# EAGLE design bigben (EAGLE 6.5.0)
AUTHOR: Brad Campbell; REV: A; TITLE: BigBen
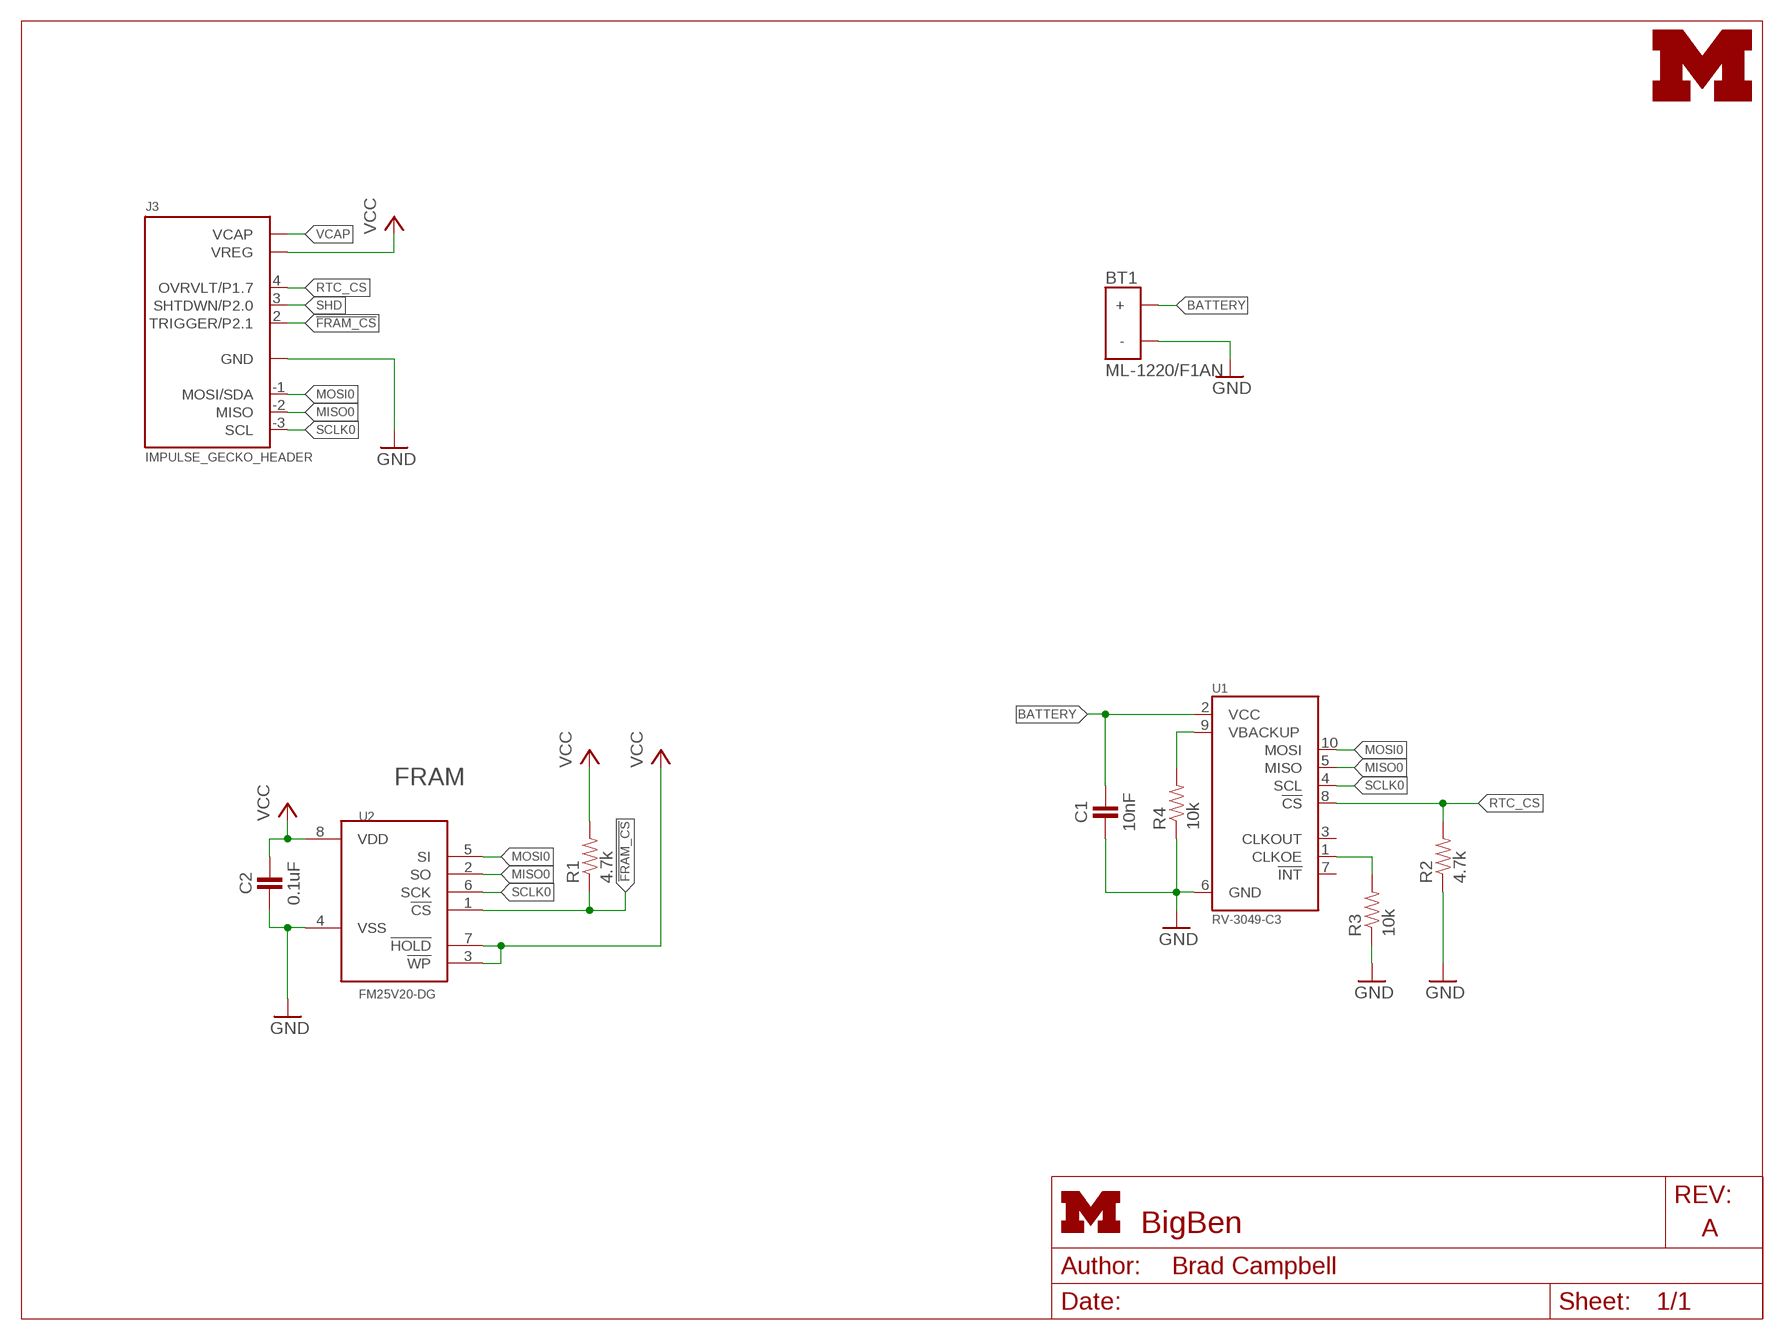
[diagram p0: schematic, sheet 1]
FRAME1 (LETTER_L): HEIGHT: 8.5in; WIDTH: 11in

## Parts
BT1  ML-1220/F1AN  [ML-1220/F1BN]
C1  10nF  CAPACITOR  [0402_CAP]
C2  0.1uF  CAPACITOR  [0402_CAP]
J3  IMPULSE_GECKO_HEADER  [HEADER1X9/0.05IN]
LOGO1  UMICH_SOLID_TINY  [UMICH_SOLID_50MIL]
R1  4.7k  RESISTOR  [0402_RES]
R2  4.7k  RESISTOR  [0402_RES]
R3  10k  RESISTOR  [0402_RES]
R4  10k  RESISTOR  [0402_RES]
U1  RV-3049-C3  [MICRO-CRYSTAL-C3]
U2  FM25V20-DG  [TDFN-8/6MM]

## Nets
!FRAM_CS: J3.2(TRIGGER/P2.1) R1.1 U2.1(!CS)
BATTERY: BT1.POS(+) C1.1 U1.2(VCC)
GND: BT1.NEG(-) C1.2 C2.2 J3.0(GND) R2.1 R3.1 R4.1 U1.6(GND) U2.4(VSS)
MISO0: J3.-2(MISO) U1.5(MISO) U2.2(SO)
MOSI0: J3.-1(MOSI/SDA) U1.10(MOSI) U2.5(SI)
N$6: R4.2 U1.9(VBACKUP)
N$7: R3.2 U1.1(CLKOE)
RTC_CS: J3.4(OVRVLT/P1.7) R2.2 U1.8(!CS)
SCLK0: J3.-3(SCL) U1.4(SCL) U2.6(SCK)
SHD: J3.3(SHTDWN/P2.0)
VCAP: J3.5(VCAP)
VCC: C2.1 J3.1(VREG) R1.2 U2.3(!WP) U2.7(!HOLD) U2.8(VDD)
Unconnected: U1.3(CLKOUT) U1.7(!INT)

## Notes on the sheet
- FRAM

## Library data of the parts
BT1 = batteries:ML-1220/F1AN: BATTERY LITH 3V RECHARGE PC PINS; DIGIKEY: P663-nd; MOUSER: 658-ML-1220/F1BN
C1 C2 = passives:CAPACITOR: 0402 Capacitor
J3 = gecko:IMPULSE_GECKO_HEADER: Header on the impulse EPIC-esque board.
LOGO1 = logos:UMICH_SOLID
R1-R4 = passives:RESISTOR: Resistor
U1 = chips:RV-3049-C3: The RV-3049-C3 is an ultra miniature Real-Time-Clock Module with embedded Crystal. This RTC has an SPI Bus (4-wire Serial- Interface) and offers temperature compensated time.
U2 = chips:FM25: Cypress FRAM; DIGIKEY: FM25V20-DGRA-ND; MOUSER: 877-FM25V20-DG

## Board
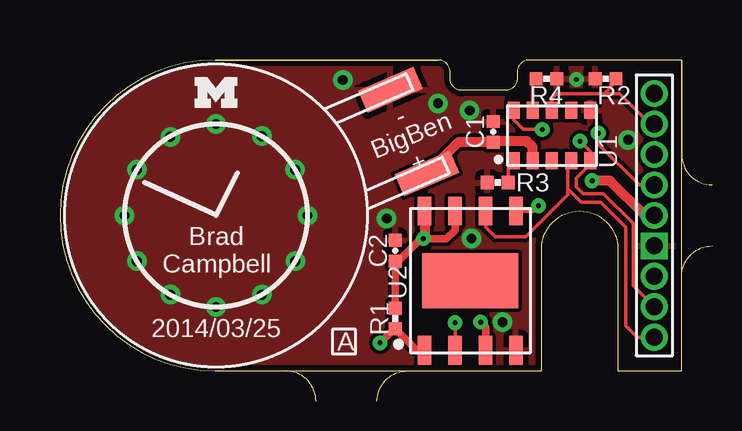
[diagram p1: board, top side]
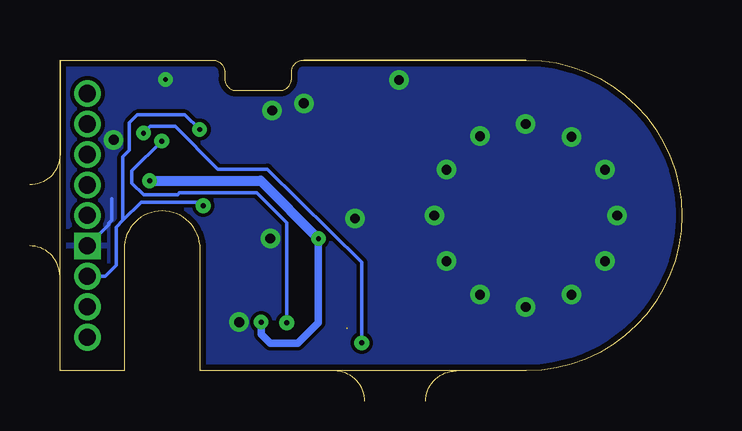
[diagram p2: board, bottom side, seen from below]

Size 25.91 x 12.95 mm. Coordinates in mm from the lower left corner, seen from the top.
Outline: 6.48,0 20.07,0 20.07,5.08 arc-180 23.24,5.08 23.24,0 25.91,0 25.91,12.95 19.56,12.95 arc90 19.05,12.45 19.05,12.19 arc-90 18.54,11.68 16.76,11.68 arc-90 16.26,12.19 16.26,12.45 arc90 15.75,12.95 6.48,12.95 arc180 6.48,0
Copper layers (1*16): Top 0.0178mm / dielectric 59mil / Bottom 0.0178mm
Design rules "sunstone-2lyr_v1.0.0.3 *": minimum track width 6mil, minimum drill 14mil, track to track 6mil, track to pad 6mil, pad to pad 6mil, via to via 6mil, smd to smd 6mil, copper to edge 10mil, drill to drill 16mil, minimum pad ring 8mil, minimum via ring 8mil, stop-mask expansion 3mil, vias tented up to drill 100mil, thermal gap 10mil
Milling: 22 lines

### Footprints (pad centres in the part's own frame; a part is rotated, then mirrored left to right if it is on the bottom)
ML-1220/F1BN = smd 2.5 x 1: NEG 8.75,1.9; POS 8.75,-1.9
0402_CAP = smd 0.536 x 0.546: 1 -0.433,0; 2 0.433,0
HEADER1X9/0.05IN = drill 0.711 pad 1.016 square: 0 -1.27,0 | drill 0.711 pad 1.016: 1 0,0; 2 1.27,0; 3 2.54,0; 4 3.81,0; 5 5.08,0; -1 -2.54,0; -2 -3.81,0; -3 -5.08,0
0402_RES = smd 0.536 x 0.546: 1 -0.433,0; 2 0.433,0
MICRO-CRYSTAL-C3 = smd 0.5 x 0.7: 1 -1.6,-1.05; 2 -0.8,-1.05; 3 0,-1.05; 4 0.8,-1.05; 5 1.6,-1.05; 6 1.6,1.05; 7 0.8,1.05; 8 0,1.05; 9 -0.8,1.05; 10 -1.6,1.05
TDFN-8/6MM = smd 0.55 x 1.2: 1 -1.905,-2.9; 2 -0.635,-2.9; 3 0.635,-2.9; 4 1.905,-2.9; 5 1.905,2.9; 6 0.635,2.9; 7 -0.635,2.9; 8 -1.905,2.9 | smd 4 x 2.3: NC 0,0

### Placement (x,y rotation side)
BT1  6.5,6.48 23.5 top
C1  18.06,9.96 90 top
C2  13.97,5 90 top
J3  24.77,6.48 90 top
LOGO1  6.5,11.61 0 top
R1  13.97,2.18 90 top
R2  22.73,12.17 0 top
R3  18.24,7.85 0 top
R4  20.27,12.17 180 top
U1  20.5,9.8 0 top
U2  17.09,3.76 0 top

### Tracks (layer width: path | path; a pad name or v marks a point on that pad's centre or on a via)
!FRAM_CS  (via drill 0.2)  (1 unrouted)
  Top 0.152: J3.2 24.13,7.75 22.43,9.45 v22.43,9.91
  Top 0.305: U2.1 14.86,0.86 R1.1 | 13.97,1.8 v13.34,1.17
  Bottom 0.152: v22.43,9.91 22.15,10.19 21.11,10.19 19.33,8.41 17.27,8.41 13.34,4.52 v13.34,1.17
BATTERY
  Top 0.406: 18.08,9.5 C1.1 | U1.2 19.7,9.33 19.46,9.58 18.11,9.58 C1.1 | C1.1 16.58,9.52 BT1.POS
GND  (via drill 0.2, 0.41)
  Bottom 0.152: J3.0 23.88,6.1 23.88,6.15 23.75,6.27 23.75,7.16
  other vias: 11.79,12.12 15.75,11.15 23.67,9.63 21.51,12.14 13.61,6.35 17.07,10.85 6.5,10.29 6.5,2.67 10.31,6.48 2.69,6.48 9.8,8.38 8.41,9.78 4.6,3.17 3.2,4.57 3.2,8.38 8.41,3.17 4.6,9.75 9.8,4.57 17.14,5.51 18.44,2.03
  pour Top: 26.42,13.72 26.42,-0.51 -0.58,-0.51 -0.58,13.72
  pour Bottom: -0.56,13.72 26.42,13.72 26.42,-0.51 -0.56,-0.51
MISO0  (via drill 0.2)
  Top 0.152: J3.-2 23.88,3.56 23.88,6.15 22.63,7.39 21.79,7.39 21.51,7.67 21.51,8.03 22.1,8.61 U1.5 22.1,9.14 v21.67,9.58 | v16.46,2.01 U2.2
  Bottom 0.152: v21.67,9.58 22.91,8.33 22.91,7.82 22.43,7.34 21.01,7.34 20.93,7.42 17.7,7.42 16.46,6.17 v16.46,2.01
MOSI0  (via drill 0.2)
  Top 0.152: U1.10 18.9,10.46 19.3,10.06 v20.09,10.06 | v19.94,6.88 19.71,6.66 U2.5
  Bottom 0.152: J3.-1 24.03,3.94 23.57,4.39 23.57,5.99 23.29,6.27 | 23.29,6.27 22.53,7.04 20.09,7.04 v19.94,6.88 | v20.09,10.06 20.7,10.67 22.68,10.67 23.01,10.34 23.01,9.2 23.29,8.91 23.29,6.27
N$6
  Top 0.152: U1.9 19.7,12.03 R4.2
N$7
  Top 0.152: U1.1 18.67,8.53 R3.2
RTC_CS
  Top 0.152: U1.8 20.5,11.35 20.7,11.56 22.68,11.56 | 22.68,11.56 23.17,12.04 R2.2 | J3.4 24.59,10.29 23.32,11.56 22.68,11.56
SCLK0
  Top 0.152: J3.-3 24.05,1.4 23.57,1.88 23.57,5.99 22.53,7.04 21.72,7.04 21.16,7.59 | 21.16,7.59 21.16,8.62 U1.4 | 21.16,7.59 21.16,7.34 19.41,5.59 18.14,5.59 17.73,5.99 U2.6
VCC  (via drill 0.2)
  Top 0.305: U2.3 17.73,1.83 v17.53,2.03 | U2.7 16.46,5.87 16.1,5.51 v15.14,5.51 15.04,5.51 14.1,4.57 C2.1 13.96,2.88 R1.2
  Top 0.406: J3.1 24.36,6.48 22.91,7.92 v22.17,7.92 | U2.8 15.19,5.56 v15.14,5.51
  Bottom 0.305: v17.53,2.03 17.53,1.52 17.14,1.14 16,1.14 15.14,2.01 v15.14,5.51
  Bottom 0.406: v22.17,7.92 17.55,7.92 v15.14,5.51

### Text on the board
tPlace: - | BigBen | + | Brad / Campbell | 2014/03/25 | A
tDocu: VCAP | OV | SHTD | TRIG | VREG | GND | MOSI | MISO | SCL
